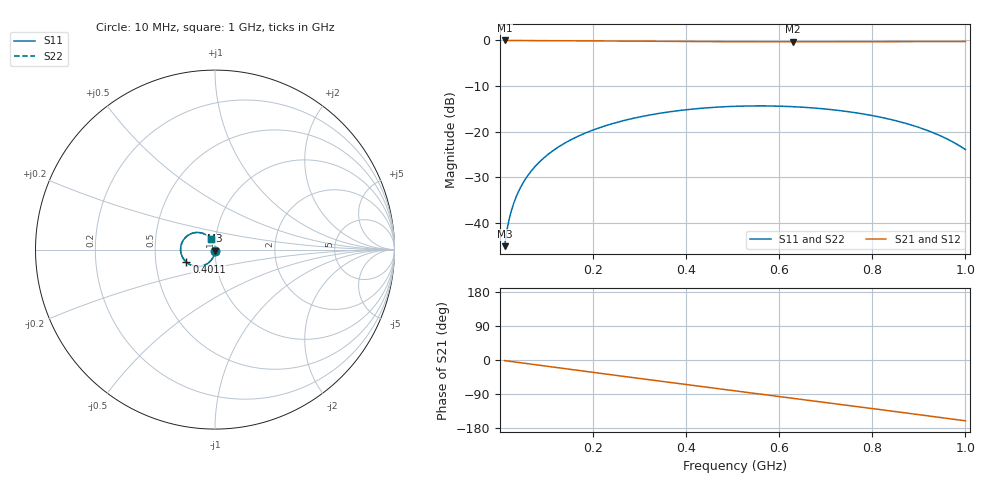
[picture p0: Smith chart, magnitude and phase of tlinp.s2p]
! AWR Design Environment (17415) Thu Oct 17 09:15:28 2024
! Document = 'TLine'
! nPorts: 2, nXvals: 201
# MHz S DB R 50
!Freq DBS11 AngS11 DBS21 AngS21 DBS12 AngS12 DBS22 AngS22
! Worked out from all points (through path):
!   201 points, 10 MHz to 1 GHz, reference 50 ohm
!   highest |S21| = -0.01 dB at 10 MHz (marker M1); lowest = -0.3 dB at 628.8 MHz (marker M2)
!   group delay of S21, straight-line fit = 443 ps
!   lowest |S11| = -45.1 dB at 10 MHz (marker M3), VSWR 1.01, Z = 50 - j0.556 ohm
!   |S11| at or under -10 dB: start of sweep to end of sweep
!   |S22| runs from -45.1 to -14.3 dB; largest |S21 - S12| = 1.7e-14
!   S11 on the Smith chart (normalised r, x): 10 MHz: 1.00, -0.01; 401.1 MHz: 0.72, -0.10; 1 GHz: 0.95, +0.11
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10  -45.10 -89.2  -0.01 -1.6  -0.01 -1.6  -45.10 -89.2
14.95  -41.61 -90.8  -0.01 -2.5  -0.01 -2.5  -41.61 -90.8
19.9  -39.13 -92.2  -0.01 -3.3  -0.01 -3.3  -39.13 -92.2
29.8  -35.64 -94.4  -0.01 -4.9  -0.01 -4.9  -35.64 -94.4
44.65  -32.14 -97.4  -0.02 -7.3  -0.02 -7.3  -32.14 -97.4
59.5  -29.67 -100.1  -0.03 -9.8  -0.03 -9.8  -29.67 -100.1
84.25  -26.70 -104.5  -0.04 -13.8  -0.04 -13.8  -26.70 -104.5
109  -24.53 -108.7  -0.05 -17.8  -0.05 -17.8  -24.53 -108.7
138.7  -22.54 -113.7  -0.07 -22.7  -0.07 -22.7  -22.54 -113.7
178.3  -20.53 -120.3  -0.09 -29.1  -0.09 -29.1  -20.53 -120.3
252.55  -17.93 -132.4  -0.14 -41.1  -0.14 -41.1  -17.93 -132.4
341.65  -15.99 -146.8  -0.20 -55.4  -0.20 -55.4  -15.99 -146.8
401.05  -15.18 -156.2  -0.23 -64.9  -0.23 -64.9  -15.18 -156.2
505  -14.44 -172.6  -0.28 -81.3  -0.28 -81.3  -14.44 -172.6
564.4  -14.35 178.1  -0.29 -90.7  -0.29 -90.7  -14.35 178.1
628.75  -14.52 168.1  -0.30 -100.9  -0.30 -100.9  -14.52 168.1
673.3  -14.80 161.2  -0.30 -107.9  -0.30 -107.9  -14.80 161.2
752.5  -15.68 148.9  -0.28 -120.5  -0.28 -120.5  -15.68 148.9
836.65  -17.26 135.9  -0.26 -134.0  -0.26 -134.0  -17.26 135.9
930.7  -20.22 121.7  -0.24 -149.2  -0.24 -149.2  -20.22 121.7
965.35  -21.83 116.8  -0.24 -154.8  -0.24 -154.8  -21.83 116.8
1000  -23.93 112.2  -0.23 -160.5  -0.23 -160.5  -23.93 112.2
